FUNCTION_BLOCK FB_CylinderTemp EXTENDS FB_Cylinder
VAR_INPUT
	lrTempCurrent		AT %I*: LREAL;
END_VAR

// =========================================================
;
// =========================================================

END_FUNCTION_BLOCK
